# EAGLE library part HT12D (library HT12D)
212 Series of Decoders Source: Datasheet
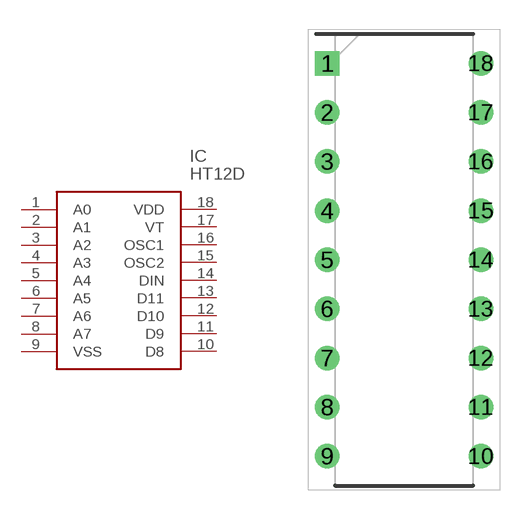
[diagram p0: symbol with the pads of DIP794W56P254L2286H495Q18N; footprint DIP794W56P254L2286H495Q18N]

Designator prefix IC

## HT12D (Description: 212 Series of Decoders; Height: 4.953mm; Manufacturer_Name: Holtek; Manufacturer_Part_Number: HT12D)  [DIP794W56P254L2286H495Q18N]
1  A0
2  A1
3  A2
4  A3
5  A4
6  A5
7  A6
8  A7
9  VSS  pwr
10  D8
11  D9
12  D10
13  D11
14  DIN  in
15  OSC2
16  OSC1
17  VT
18  VDD  pwr

## Footprint DIP794W56P254L2286H495Q18N (pad centres in mm)
18-pin DIP (300mil)
drill 0.759 pad 1.159 square: 1 -3.969,10.16
drill 0.759 pad 1.159: 2 -3.969,7.62; 3 -3.969,5.08; 4 -3.969,2.54; 5 -3.969,0; 6 -3.969,-2.54; 7 -3.969,-5.08; 8 -3.969,-7.62; 9 -3.969,-10.16; 10 3.969,-10.16; 11 3.969,-7.62; 12 3.969,-5.08; 13 3.969,-2.54; 14 3.969,0; 15 3.969,2.54; 16 3.969,5.08; 17 3.969,7.62; 18 3.969,10.16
